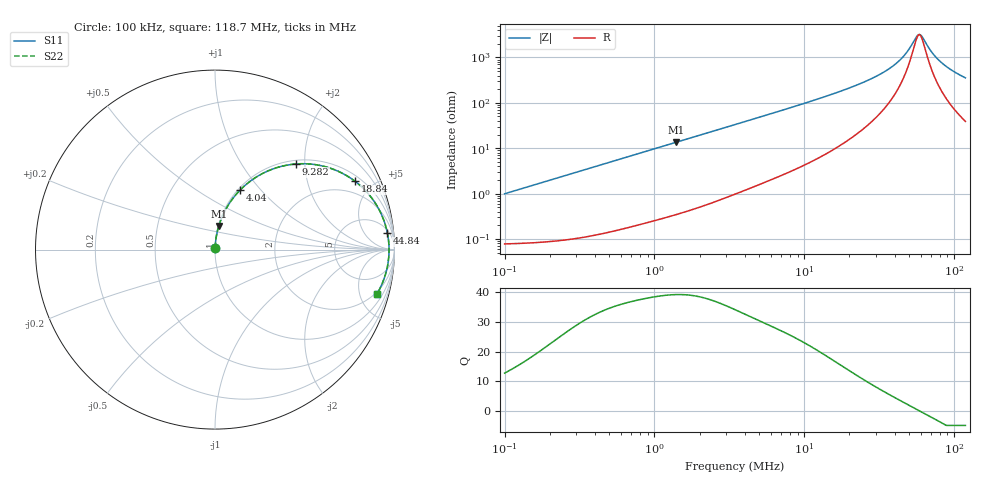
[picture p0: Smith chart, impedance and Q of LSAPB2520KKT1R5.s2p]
! LSAPB2520KKT1R5  S-PARAMETER MODEL  ( General Type )
! Model Generated by TAIYO YUDEN Corporation (http://www.ty-top.com)
! Version 2.0
! TAIYO YUDEN Control No. 20210629
! Copyright(c) 2015 TAIYO YUDEN CO.,LTD. All Rights Reserved.
! Product Description (link to TY-COMPAS)
! https://ds.yuden.co.jp/TYCOMPAS/or/detail?pn=LSAPB2520KKT1R5M&u=M
! Products Name : Inductors
! Characteristics :
!  Inductance : 1.5 uH , SRF(min) : -Hz , DC Resistance(max) : 0.078 Ohm
!  Rated Current : Saturation :3000 mA , Temp Rise : 2400 mA (40 degC)
!  Case Size : 2.5 x 2.0 / 0.098 x 0.079 [mm/inch] , Thickness : 1 / 0.039 [mm/inch]
!  (Conditions: Temperature = 25 degC , DC Bias Current/Voltage = 0A / 0V)
! External Node Assignments :
!  1  o---GGG---o  2
! GND o---------o GND
! Frequency Range : 0.1MHz  -  118.695536MHz  [ 402 STEP ]
# MHz S RI R 50
! Freq[MHz].  S11 Real  S11 Imag  S21 Real  S21 Imag  S12 Real  S12 Imag  S22 Real  S22 Imag
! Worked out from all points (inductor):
!   401 points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, 100 kHz to 118.7 MHz, reference 50 ohm
!   read as one part in series: L = 1.57 uH near 103.6 kHz
!   highest Q = 39.3 at 1.397 MHz (marker M1), where L = 1.54 uH
!   self-resonance near 58.46 MHz
!   S11 on the Smith chart (normalised r, x): 100 kHz: 1.00, +0.02; 4.04 MHz: 1.02, +0.78; 9.282 MHz: 1.08, +1.80; 18.84 MHz: 1.28, +3.95; 44.84 MHz: 7, +19; 118.7 MHz: 1.78, -7.07
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0.1  0.000875 0.00987  0.9991 -0.00987  0.9991 -0.00987  0.000875 0.00987
0.327316  0.0021 0.0321  0.9979 -0.0321  0.9979 -0.0321  0.0021 0.0321
1.07136  0.0133 0.1025  0.9867 -0.1025  0.9867 -0.1025  0.0133 0.1025
1.397098  0.0213 0.1322  0.9787 -0.1322  0.9787 -0.1322  0.0213 0.1322
2.293175  0.0518 0.2087  0.9482 -0.2087  0.9482 -0.2087  0.0518 0.2087
3.445222  0.106 0.2935  0.894 -0.2935  0.894 -0.2935  0.106 0.2935
4.040099  0.1387 0.3306  0.8613 -0.3306  0.8613 -0.3306  0.1387 0.3306
6.069766  0.2616 0.4223  0.7384 -0.4223  0.7384 -0.4223  0.2616 0.4223
9.281924  0.4503 0.477  0.5497 -0.477  0.5497 -0.477  0.4503 0.477
11.27678  0.5482 0.4749  0.4518 -0.4749  0.4518 -0.4749  0.5482 0.4749
18.84002  0.7807 0.3803  0.2193 -0.3803  0.2193 -0.3803  0.7807 0.3803
27.80836  0.8951 0.2559  0.1049 -0.2559  0.1049 -0.2559  0.8951 0.2559
36.91074  0.9426 0.158  0.0574 -0.158  0.0574 -0.158  0.9426 0.158
44.84352  0.9609 0.0908  0.0391 -0.0908  0.0391 -0.0908  0.9609 0.0908
48.99256  0.9658 0.0604  0.0342 -0.0604  0.0342 -0.0604  0.9658 0.0604
56.44413  0.9696 0.012  0.0304 -0.012  0.0304 -0.012  0.9696 0.012
59.52193  0.9698 -0.00616  0.0302 0.00616  0.0302 0.00616  0.9698 -0.00616
61.66649  0.9695 -0.0183  0.0305 0.0183  0.0305 0.0183  0.9695 -0.0183
71.04572  0.9653 -0.0668  0.0347 0.0668  0.0347 0.0668  0.9653 -0.0668
80.41563  0.9575 -0.1095  0.0425 0.1095  0.0425 0.1095  0.9575 -0.1095
95.98456  0.9389 -0.1709  0.0611 0.1709  0.0611 0.1709  0.9389 -0.1709
118.6955  0.9037 -0.245  0.0963 0.245  0.0963 0.245  0.9037 -0.245
